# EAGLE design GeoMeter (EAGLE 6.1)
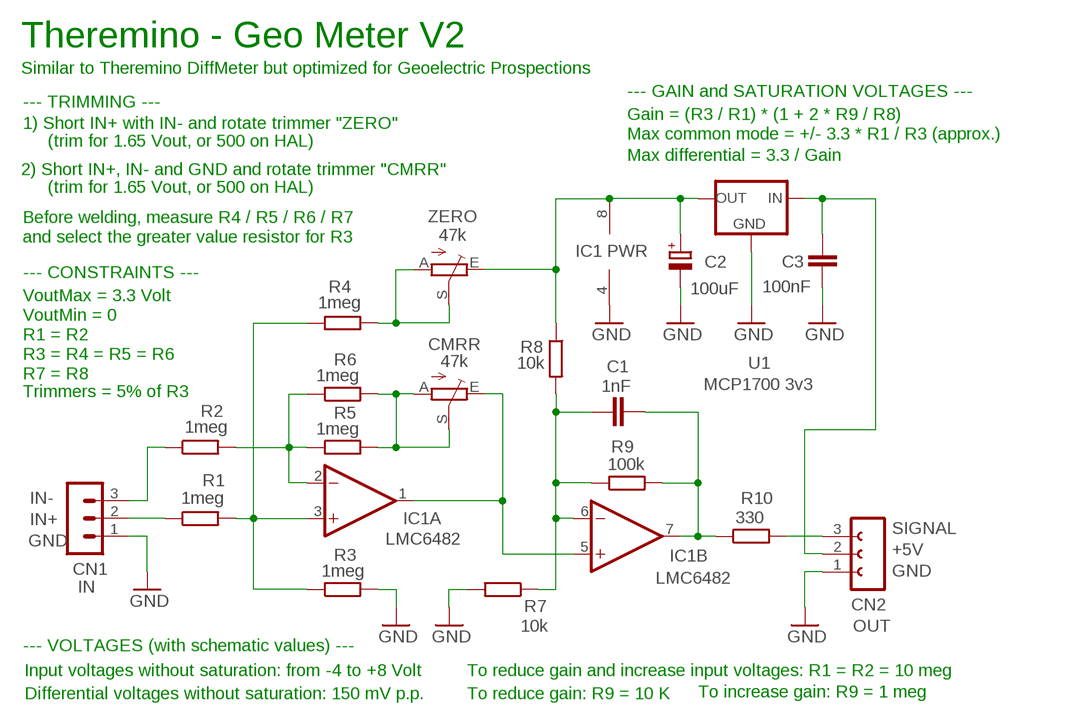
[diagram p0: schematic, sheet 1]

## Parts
C1  1nF  C-EU025-024X044  [C025-024X044]
C2  100uF  CPOL-EUE2-5B  [E2-5B]
C3  100nF  C-EU025-024X044  [C025-024X044]
CMRR  47k  TRIMMERTRIM_M2  [TRIM_M2]
CN1  IN  MA03-1N  [MA03-1]
CN2  OUT  FE03-1"  [FE03-1]
IC1  LMC6482  TL072P  [DIL08]
R1  1meg  R-EU_0204/5  [0204/5]
R2  1meg  R-EU_0204/5  [0204/5]
R3  1meg  R-EU_0204/5  [0204/5]
R4  1meg  R-EU_0204/5  [0204/5]
R5  1meg  R-EU_0204/5  [0204/5]
R6  1meg  R-EU_0204/5  [0204/5]
R7  10k  R-EU_0204/5  [0204/5]
R8  10k  R-EU_0204/5  [0204/5]
R9  100k  R-EU_0204/5  [0204/5]
R10  330  R-EU_0204/5  [0204/5]
U1  MCP1700 3v3  MCP1700L1  [TO92L1]
ZERO  47k  TRIMMERTRIM_M2  [TRIM_M2]

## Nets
GND: C2.- C3.2 CN1.1 CN2.1 IC1.4(P:V-) R3.2 R7.2 U1.3(GND)
N$1: IC1.2(A:-IN) R2.2 R5.1 R6.1
N$2: C1.1 IC1.6(B:-IN) R7.1 R8.2 R9.1
N$3: R4.2 ZERO.A ZERO.S
N$4: IC1.3(A:+IN) R1.2 R3.1 R4.1
N$5: C1.2 IC1.7(B:OUT) R9.2 R10.1
N$6: CMRR.E IC1.1(A:OUT) IC1.5(B:+IN)
N$7: CN2.3 R10.2
N$8: C3.1 CN2.2 U1.2(IN)
N$9: CN1.2 R1.1
N$10: C2.+ IC1.8(P:V+) R8.1 U1.1(OUT) ZERO.E
N$11: CN1.3 R2.1
N$16: CMRR.A CMRR.S R5.2 R6.2

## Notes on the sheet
- Theremino - Geo Meter V2
- Similar to Theremino DiffMeter but optimized for Geoelectric Prospections
- --- GAIN and SATURATION VOLTAGES ---
- --- TRIMMING ---
- Gain = (R3 / R1) * (1 + 2 * R9 / R8)
- 1) Short IN+ with IN- and rotate trimmer "ZERO"
- Max common mode = +/- 3.3 * R1 / R3 (approx.)
- (trim for 1.65 Vout, or 500 on HAL)
- Max differential = 3.3 / Gain
- 2) Short IN+, IN- and GND and rotate trimmer "CMRR"
- (trim for 1.65 Vout, or 500 on HAL)
- Before welding, measure R4 / R5 / R6 / R7
- and select the greater value resistor for R3
- IC1 PWR
- --- CONSTRAINTS ---
- VoutMax = 3.3 Volt
- VoutMin = 0
- R1 = R2
- R3 = R4 = R5 = R6
- R7 = R8
- Trimmers = 5% of R3
- IN-
- IN+
- SIGNAL
- GND
- +5V
- GND
- --- VOLTAGES (with schematic values) ---
- Input voltages without saturation: from -4 to +8 Volt | To reduce gain and increase input voltages: R1 = R2 = 10 meg
- Differential voltages without saturation: 150 mV p.p. | To reduce gain: R9 = 10 K | To increase gain: R9 = 1 meg

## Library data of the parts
C1 C3 = 00-LIVIO:C-EU: CAPACITOR, European symbol
C2 = 00-LIVIO:CPOL-EU: POLARIZED CAPACITOR, European symbol
CMRR ZERO = 00-LIVIO:TRIMMER: Horizzontal and Vertical trimmers
CN1 = 03-con-lstb-M:MA03-1: PIN HEADER
CN2 = 02-con-lsta-F:FE03-1: FEMALE HEADER
IC1 = linear:TL072: OP AMP
R1-R10 = 00-LIVIO:R-EU_: RESISTOR, European symbol
U1 = 00-LIVIO:MCP1700: Linear regulator Quescient courrent 1.8uA Input 2.3v to 6v Output 1.2v 1.8v 2.5v 3.0v 3.3v 5.0v

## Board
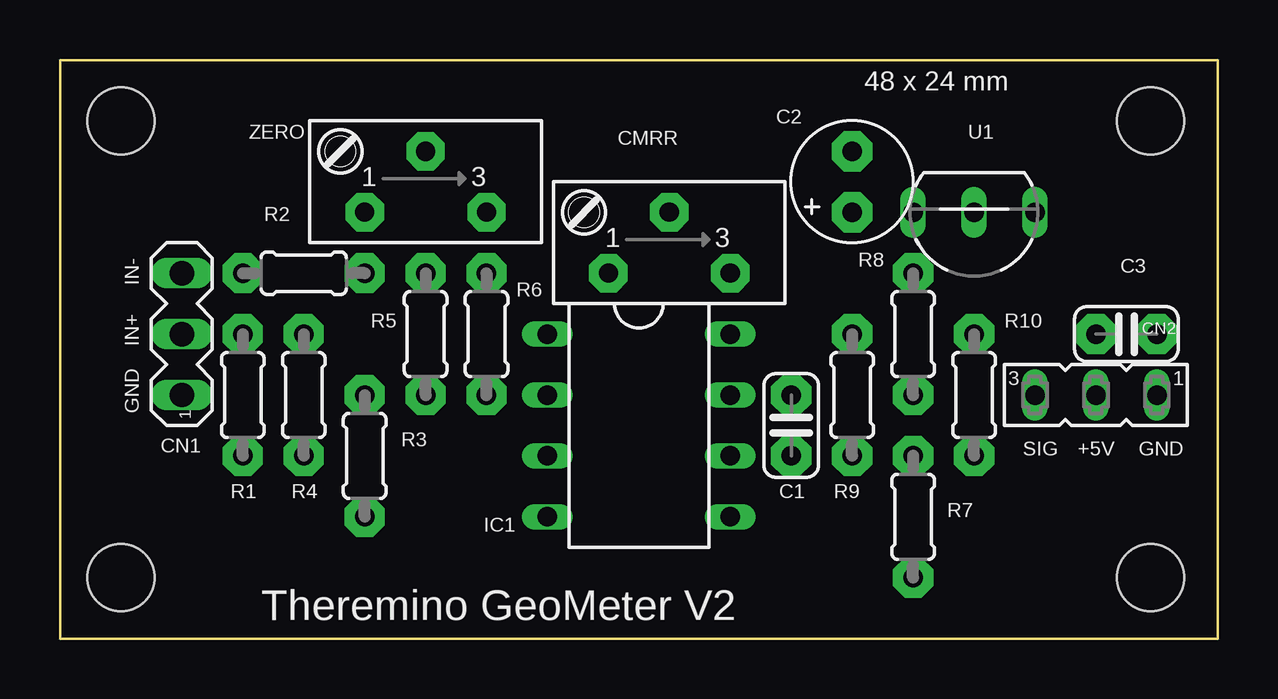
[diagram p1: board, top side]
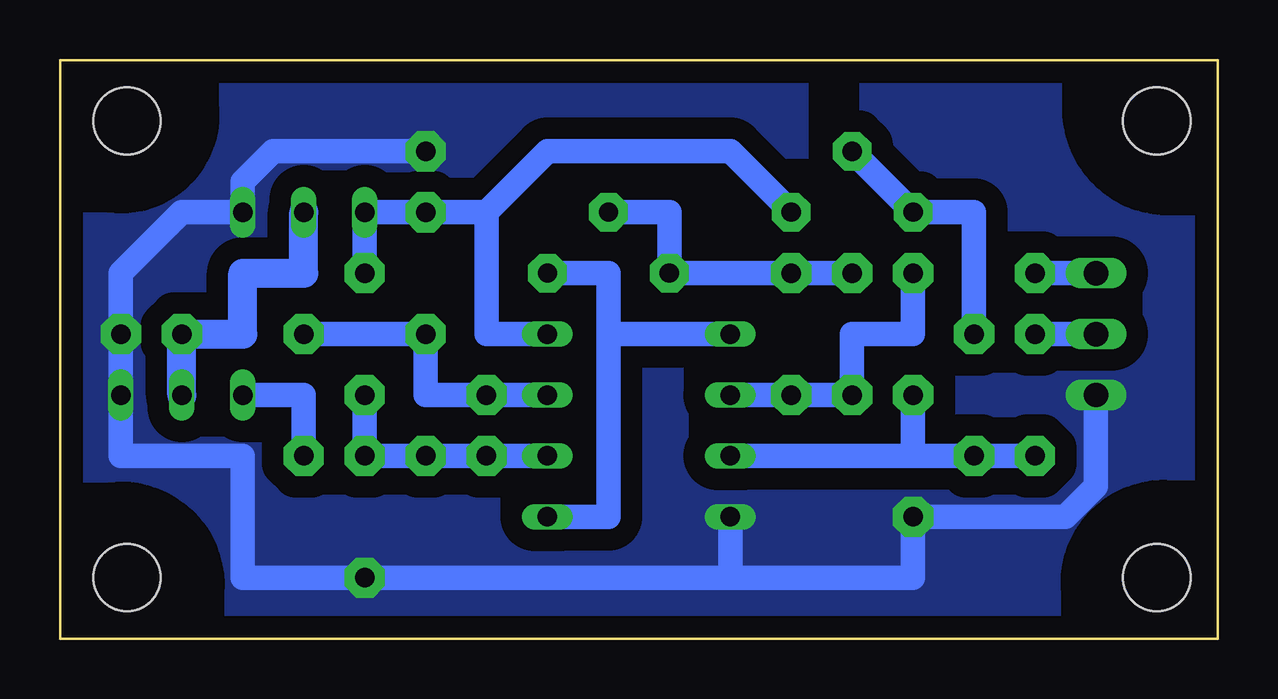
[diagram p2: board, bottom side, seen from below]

Size 48.26 x 24.13 mm. Coordinates in mm from the lower left corner, seen from the top.
Outline: 0,0 48.26,0 48.26,24.13 0,24.13 0,0
Copper layers (1*16): Top 0.035mm / dielectric 1.5mm / Bottom 0.035mm
Design rules: minimum track width 10mil, minimum drill 31mil, track to track 31mil, track to pad 31mil, pad to pad 31mil, via to via 31mil, smd to smd 31mil, copper to edge 31mil, drill to drill 8mil, minimum pad ring 5mil, minimum via ring 8mil, stop-mask expansion 4mil, vias tented up to drill 0mil, thermal gap 47mil
Holes 2.8 mm at 2.54,21.59 45.47,21.59 45.47,2.54 2.54,2.54
bRestrict: 5 lines

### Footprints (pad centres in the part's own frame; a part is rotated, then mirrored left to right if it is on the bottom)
C025-024X044 = drill 0.813 pad 1.676 octagon: 1 -1.27,0; 2 1.27,0
E2-5B = drill 0.813 pad 1.676 octagon: + -1.27,0; - 1.27,0
TRIM_M2 = drill 0.8 pad 1.6 octagon: A 2.54,2.54; E -2.54,2.54; S 0,0
MA03-1 = drill 1.016 long: 1 -2.54,0; 2 0,0; 3 2.54,0
FE03-1 = drill 0.813 long: 1 -2.54,0; 2 0,0; 3 2.54,0
DIL08 = drill 0.813 long: 1 -3.81,-3.81; 2 -1.27,-3.81; 3 1.27,-3.81; 4 3.81,-3.81; 5 3.81,3.81; 6 1.27,3.81; 7 -1.27,3.81; 8 -3.81,3.81
0204/5 = drill 0.813 pad 1.676 octagon: 1 -2.54,0; 2 2.54,0
TO92L1 = drill 0.813 long: 1 2.54,0; 2 0,0; 3 -2.54,0

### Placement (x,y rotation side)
C1  30.48,8.89 90 top
C2  33.02,19.05 90 top
C3  44.45,12.7 0 top
CMRR  25.4,17.78 180 top
CN1  5.08,12.7 90 top
CN2  43.18,10.16 180 top
IC1  24.13,8.89 270 top
R1  7.62,10.16 270 top
R2  10.16,15.24 0 top
R3  12.7,7.62 270 top
R4  10.16,10.16 90 top
R5  15.24,12.7 90 top
R6  17.78,12.7 90 top
R7  35.56,5.08 270 top
R8  35.56,12.7 270 top
R9  33.02,10.16 90 top
R10  38.1,10.16 270 top
U1  38.1,17.78 180 top
ZERO  15.24,20.32 180 top

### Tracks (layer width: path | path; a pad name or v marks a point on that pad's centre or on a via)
GND
  Bottom 1.016: C2.- 38.1,20.32 39.37,20.32 40.64,19.05 U1.3 43.18,17.78 45.72,15.24 C3.2 CN2.1 45.72,8.64 45.72,7.62 40.64,7.62 40.64,2.54 R7.2 20.32,2.54 | 20.32,2.54 IC1.4 | 20.32,2.54 12.7,2.54 R3.2 6.35,5.08 5.08,6.35 CN1.1
  pour Bottom (isolate 0.9, rank 6, no thermals): -1,-1 49.01,-1 49.01,25.13 -1,25.13
N$1
  Bottom 1.016: IC1.2 R6.1 R5.1 15.24,12.7 12.7,12.7 R2.2
N$2
  Bottom 1.016: IC1.6 C1.1 R7.1 | R7.1 R9.1 R7.1 | R8.2 R7.1
N$3
  Bottom 1.016: ZERO.S ZERO.A 10.16,17.78 10.16,12.95 R4.2
N$4
  Bottom 1.016: IC1.3 12.7,7.62 | R1.2 R4.1 12.7,7.62 | 12.7,7.62 R3.1 12.7,7.62
N$5
  Bottom 1.016: IC1.7 C1.2 33.02,10.16 R9.2 R10.1
N$6
  Bottom 1.016: CMRR.E 25.4,15.24 25.4,12.7 | 25.4,12.7 25.4,5.08 IC1.5 | IC1.1 25.4,12.7
N$7
  Bottom 1.016: CN2.3 38.1,10.16 R10.2
N$8
  Bottom 1.2: CN2.2 C3.1 40.64,12.7 40.64,15.24 38.1,15.24 U1.2
N$9
  Bottom 1.016: CN1.2 R1.1
N$10
  Bottom 1.016: ZERO.E 20.32,20.32 27.94,20.32 30.48,17.78 | 30.48,17.78 C2.+ U1.1 R8.1 | IC1.8 30.48,12.7 30.48,17.78
N$11
  Bottom 1.016: CN1.3 R2.1
N$16
  Bottom 1.016: CMRR.S 22.86,17.78 CMRR.A 20.32,15.24 R6.2 R5.2

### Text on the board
tNames: 48 x 24 mm | IN- | IN+ | GND | SIG | +5V | GND | Theremino GeoMeter V2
